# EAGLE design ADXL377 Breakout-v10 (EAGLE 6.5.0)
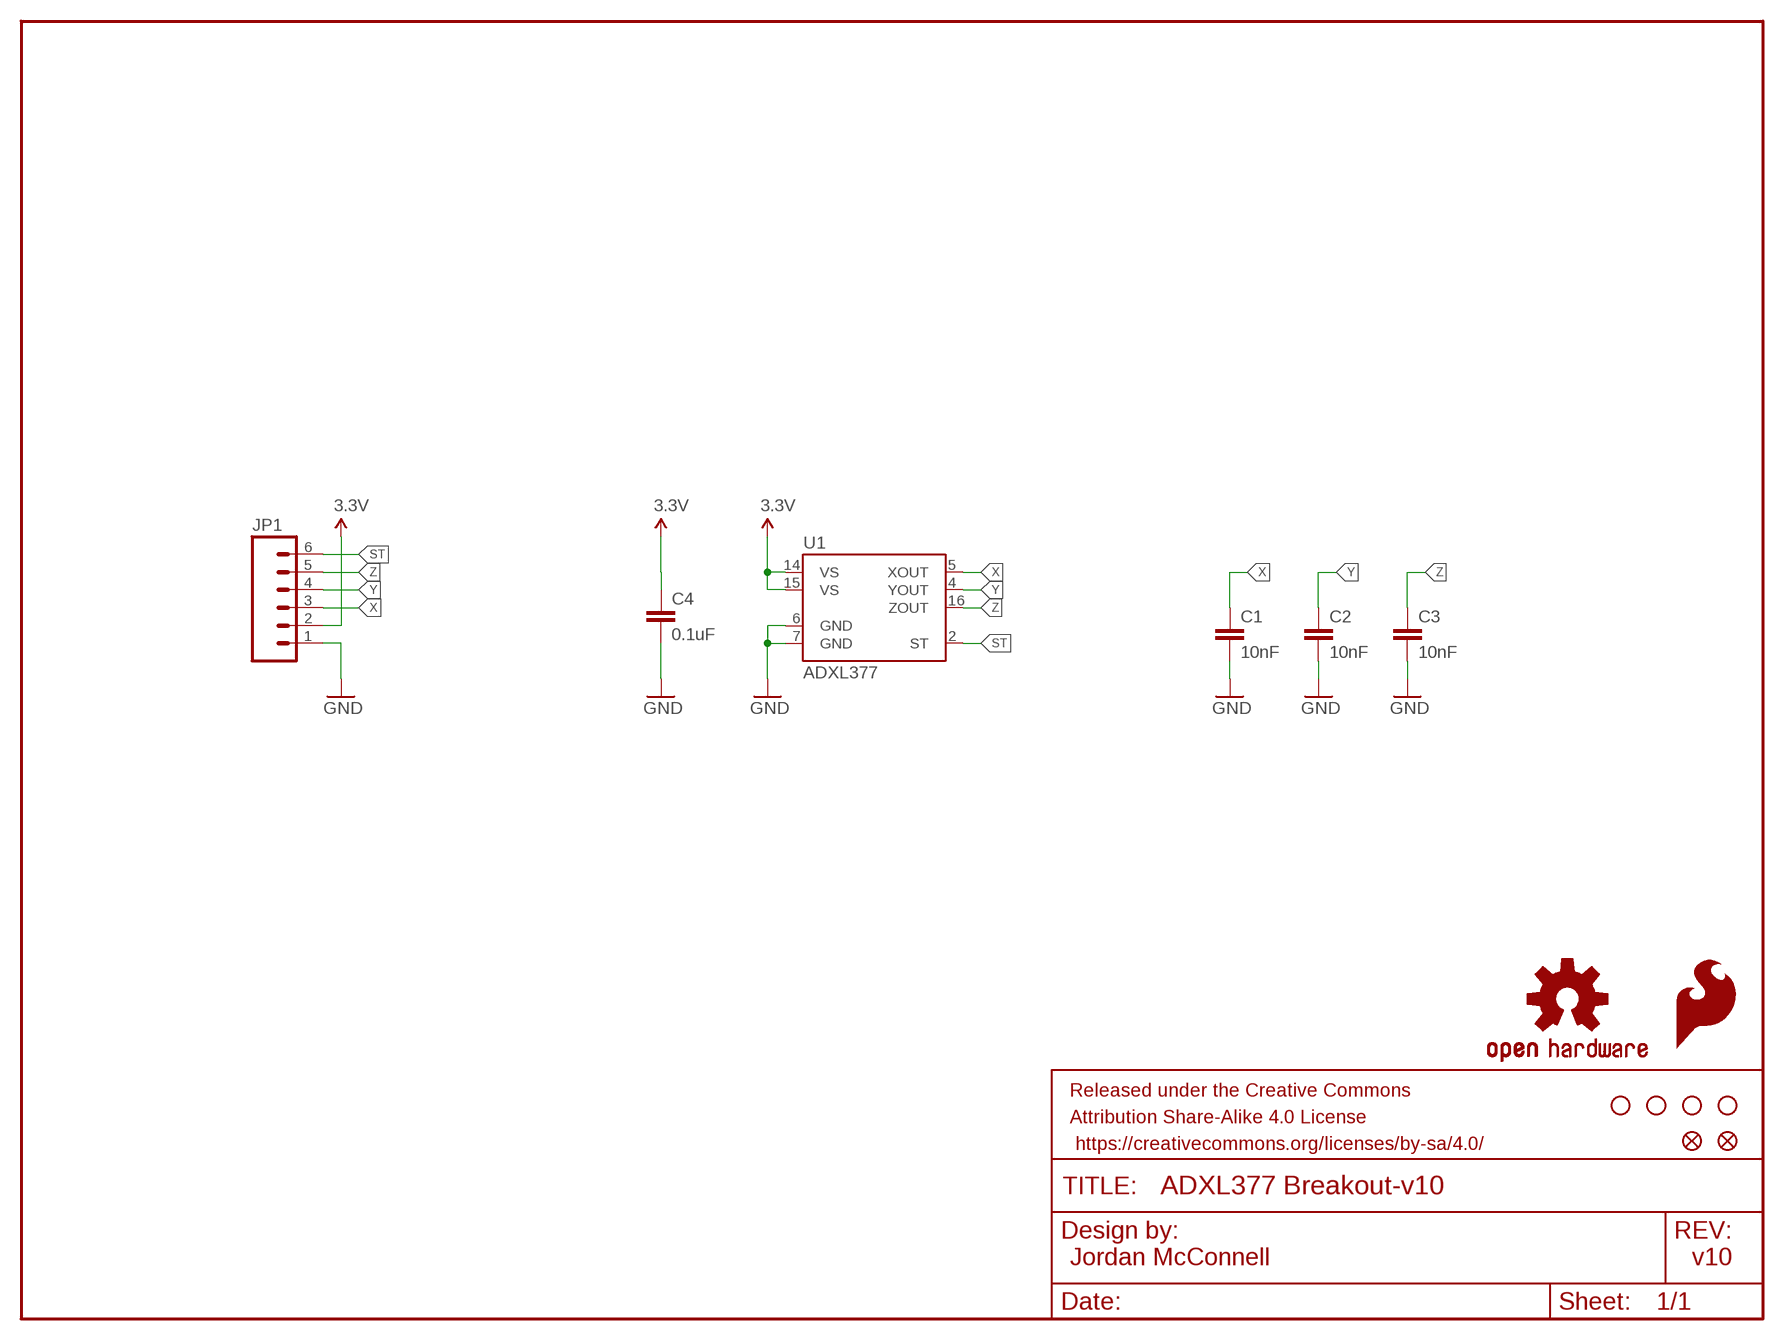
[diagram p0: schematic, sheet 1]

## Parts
C1  10nF  10NF/10000PF-50V-10%(0603)  [0603-CAP]
C2  10nF  10NF/10000PF-50V-10%(0603)  [0603-CAP]
C3  10nF  10NF/10000PF-50V-10%(0603)  [0603-CAP]
C4  0.1uF  0.1UF-25V(+80/-20%)(0603)  [0603-CAP]
FID1  FIDUCIAL1X2  [FIDUCIAL-1X2]
FID2  FIDUCIAL1X2  [FIDUCIAL-1X2]
FRAME1  FRAME-LETTER  [CREATIVE_COMMONS]
JP1  M06SIP  [1X06]
LOGO1  SFE_LOGO_FLAME.1_INCH  [SFE_LOGO_FLAME_.1]
LOGO2  OSHW-LOGOS  [OSHW-LOGO-S]
STANDOFF1  STAND-OFF  [STAND-OFF]
STANDOFF2  STAND-OFF  [STAND-OFF]
STANDOFF3  STAND-OFF  [STAND-OFF]
STANDOFF4  STAND-OFF  [STAND-OFF]
U1  ADXL377  [LFCSP_LQ-16]

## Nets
3.3V: C4.1 JP1.2 U1.14(VS) U1.15(VS)
GND: C1.2 C2.2 C3.2 C4.2 JP1.1 U1.6(GND) U1.7(GND)
ST: JP1.6 U1.2(ST)
X: C1.1 JP1.3 U1.5(XOUT)
Y: C2.1 JP1.4 U1.4(YOUT)
Z: C3.1 JP1.5 U1.16(ZOUT)

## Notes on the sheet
- Jordan McConnell | v10

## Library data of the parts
C1-C3 = SparkFun-Capacitors:10NF/10000PF-50V-10%(0603): CAP-00867; PROD_ID: CAP-00867
C4 = SparkFun-Capacitors:0.1UF-25V(+80/-20%)(0603): CAP-00810; PROD_ID: CAP-00810
FID1 FID2 = SparkFun-Aesthetics:FIDUCIAL: Fiducial Alignment Points
FRAME1 = SparkFun-Aesthetics:FRAME-LETTER: Schematic Frame
JP1 = SparkFun-Connectors:M06: Header 6 Standard 6-pin 0.1" header. Use with straight break away headers (SKU : PRT-00116), right angle break away headers (PRT-00553), swiss pins (PRT-00743), machine pins (PRT-00117), and female headers (PRT-00115). Molex polarized connector foot print use with SKU : PRT-08094 with associated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
LOGO1 = SparkFun-Aesthetics:SFE_LOGO_FLAME: SFE Logo, flame only
LOGO2 = SparkFun-Aesthetics:OSHW-LOGO: Open Source Hardware Logo This logo indicates the piece of hardware it is found on incorporates a OSHW license and/or adheres to the definition of open source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
STANDOFF1-STANDOFF4 = SparkFun-Electromechanical:STAND-OFF: #4 Stand Off
U1 = SparkFun-Sensors:ADXL377: ADXL377 Low Power 3-Axis ±200 g Accelerometer with Analog Output.

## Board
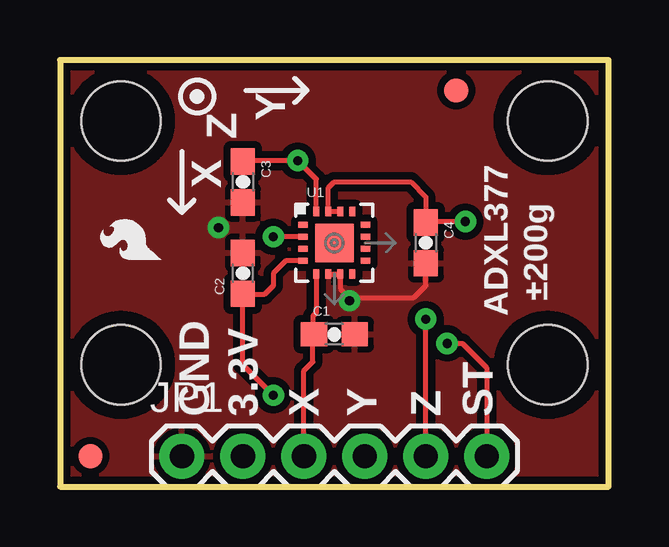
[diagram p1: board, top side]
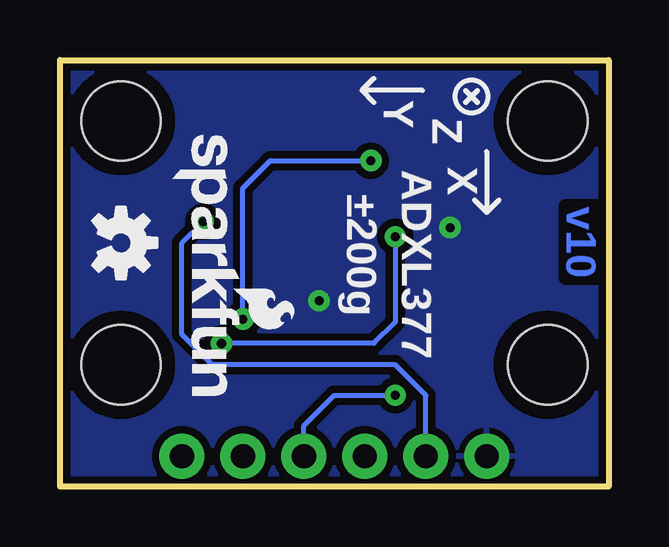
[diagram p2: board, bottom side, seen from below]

Size 22.86 x 17.78 mm. Coordinates in mm from the lower left corner, seen from the top.
Outline: 0,0 22.86,0 22.86,17.78 0,17.78 0,0
Copper layers (1*16): Top 0.035mm / dielectric 1.5mm / Bottom 0.035mm
Design rules "SparkFun": minimum track width 8mil, minimum drill 20mil, track to track 8mil, track to pad 8mil, pad to pad 8mil, via to via 8mil, smd to smd 8mil, copper to edge 8mil, drill to drill 8mil, minimum pad ring 12mil, minimum via ring 10mil, stop-mask expansion 4mil, vias tented up to drill 20mil, thermal gap 10mil

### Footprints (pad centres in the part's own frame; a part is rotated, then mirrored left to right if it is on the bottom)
0603-CAP = smd 1.1 x 1: 1 -0.85,0; 2 0.85,0
FIDUCIAL-1X2 = smd 1 x 1: 1 0,0
1X06 = drill 1.016 pad 1.88: 1 0,0; 2 2.54,0; 3 5.08,0; 4 7.62,0; 5 10.16,0; 6 12.7,0
STAND-OFF = hole 3.302: 0,0
LFCSP_LQ-16 = smd 0.4 x 0.25: 1 -1.3,0.75; 2 -1.3,0.25; 3 -1.3,-0.25; 4 -1.3,-0.75; 9 1.3,-0.75; 10 1.3,-0.25; 11 1.3,0.25; 12 1.3,0.75 | smd 0.25 x 0.4: 5 -0.75,-1.3; 6 -0.25,-1.3; 7 0.25,-1.3; 8 0.75,-1.3; 13 0.75,1.3; 14 0.25,1.3; 15 -0.25,1.3; 16 -0.75,1.3 | smd 1.6 x 1.6: EXP 0,0

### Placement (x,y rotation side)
C1  11.43,6.35 0 top
C2  7.62,8.89 90 top
C3  7.62,12.7 270 top
C4  15.24,10.16 270 top
FID1  16.51,16.51 0 top
FID2  1.27,1.27 0 top
FRAME1  not placed on the board
JP1  5.08,1.27 0 top
LOGO1  4.57,9.14 90 top
LOGO2  20.32,10.16 270 bottom
LOGO3  SFE_LOGO_NAME_FLAME.1_INCH  [SFE_LOGO_NAME_FLAME_.1]  18.29,15.11 270 bottom
STANDOFF1  20.32,15.24 0 top
STANDOFF2  2.54,5.08 0 top
STANDOFF3  2.54,15.24 0 top
STANDOFF4  20.32,5.08 0 top
U1  11.43,10.16 0 top

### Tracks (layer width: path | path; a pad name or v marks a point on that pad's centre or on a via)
3.3V  (via drill 0.38)
  Top 0.203: U1.14 U1.15 11.18,12.45 11.43,12.7 14.61,12.7 15.24,12.06 C4.1 15.28,11.05 v16.89,11.05
  Bottom 0.203: JP1.2 7.62,3.81 8.89,5.08 16.51,5.08 17.78,6.35 17.78,10.16 v16.89,11.05
GND  (via drill 0.38)
  Top 0.203: U1.6 U1.7 11.68,8.26 12.06,7.87 14.73,7.87 15.24,8.38 C4.2
  other vias: 6.6,10.79 12.06,7.75
  pour Bottom (isolate 0.305): 0,17.78 22.86,17.78 22.86,0 0,0
  pour Top (isolate 0.305): 0,0 0,17.78 22.86,17.78 22.86,0
ST  (via drill 0.38)
  Top 0.203: U1.2 v8.89,10.41 | v16.13,5.97 16.76,5.97 17.78,4.95 JP1.6
  Bottom 0.203: v8.89,10.41 8.89,6.86 9.78,5.97 v16.13,5.97
X
  Top 0.203: JP1.3 10.16,4.83 10.54,5.21 10.54,6.31 C1.1 10.54,6.39 10.54,7.11 10.68,7.25 U1.5
Y  (via drill 0.38)
  Top 0.203: v8.89,3.81 7.62,5.08 C2.1 7.66,8 8.51,8 8.89,8.38 8.89,8.89 9.41,9.41 U1.4
  Bottom 0.203: JP1.4 12.7,2.54 11.43,3.81 v8.89,3.81
Z  (via drill 0.38)
  Top 0.203: U1.16 10.68,12.81 v9.91,13.59 8.89,13.59 | 8.89,13.59 7.66,13.59 | 7.66,13.59 C3.1 7.66,13.59 | JP1.5 v15.24,6.99 | 8.89,13.59 7.66,13.59
  Bottom 0.203: v15.24,6.99 15.24,12.45 14.1,13.59 v9.91,13.59

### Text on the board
Bottom: v10
tPlace: Y | Z | X | ±200g | ADXL377 | GND | 3.3V | X | Y | Z | ST
bPlace: Y | Z | X | ADXL377 | ±200g
tNames: Jordan McConnell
